|   stm32f401_d_e_wlcsp49 IBIS Model
[IBIS ver]   4.2
[File name]  stm32f401_d_e_wlcsp49.ibs
[File Rev]   1.0
[Date]   09-06-2015
[Source] Data Created at STMicroelectronics
[Notes]   File originated from ELDO simulations.
[Disclaimer]  This information is for modeling purpose only and is
   not guaranted. The information is subject to change without
   notice.
[Copyright] Copyright 2015 STMicroelectronics Inc.
[Component] stm32f401_d_e_wlcsp49
[Manufacturer] STMicroelectronics
[Package]
| variable   typ   min   max
R_pkg   0.0   NA   NA
L_pkg   0.0H   NA   NA
C_pkg   0.0F   NA   NA
[Pin]   signal_name   model_name   R_pin   L_pin   C_pin
A1 PA14 io8p_arsudq_ft
A2 PA15 io8p_arsudq_ft
A3 PB3 io8p_arsudq_i2cin_ft
A4 PB4 io8p_arsudq_i2cin_ft
A5 BOOT0 vpp_test_hv
A6 VSS gnd
A7 VDD power
B1 VSS gnd
B2 VDD power
B3 PA13 io8p_arsudq_ft
B4 PB5 io8p_ar3wsudq_ft
B5 PB8 io8p_arsudq_i2cin_ft
B6 PDR_ON io8p_arsudq_ft_v33
B7 VBAT power
C1 PA11 io8usb_lsfs_otg_ft
C2 PA10 io8usb_id_otg_ft
C3 PA12 io8usb_lsfs_otg_ft
C4 PB6 io8p_arsudq_i2cin_ft
C5 PB9 io8p_arsudq_i2cin_ft
C6 PC15-OSC32_OUT io8p_arsudq_ft
C7 PC14-OSC32_IN io8p_arwsudq_ft
D1 PA8 io8p_arsudq_i2cin_ft
D2 PA9 io8usb_vbus_otg_ft
D3 VSS gnd
D4 PB7 io8p_arsudq_i2cin_ft
D5 PC13-ANTI_TAMP io8p_arwsudq_ft_v33
D6 PH1-OSC_OUT io8p_arsudq_ft
D7 PH0-OSC_IN io8p_arsudq_ft
E1 PB15 io8p_arsudq_ft
E2 PB12 io8p_arsudq_ft
E3 PB10 io8p_arsudq_i2cin_ft
E4 PA3 io8p_arwsudq_ft
E5 PA2 io8p_arwsudq_ft
E6 VSS gnd
E7 NRST ioreset_ft_v33
F1 PB14 io8p_arsudq_ft
F2 VDD power
F3 PA7 io8p_arwsudq_ft
F4 PA6 io8p_ar3wsudq_ft
F5 PA5 io8p_ar3wsudq_ft
F6 PA0-WKUP io8p_arwsudq_ft_v33
F7 VDDA power
G1 PB13 io8p_arsudq_ft
G2 VCAP1 power
G3 PB2 io8p_arwsudq_ft
G4 PB1 io8p_ar3wsudq_ft
G5 PB0 io8p_ar3wsudq_ft
G6 PA4 io8p_ar3wsudq_ft
G7 PA1 io8p_arwsudq_ft
[Diff Pin]   inv_pin   vdiff   tdelay_typ  tdelay_min  tdelay_max
C1 C3 200mV   NA   NA   NA
[Model Selector] io8p_ar3wsudq_ft
io8p00_ar3wsudq_ft_pd_lv  "SPEED00 1P8V, PD=40kOhm"
io8p00_ar3wsudq_ft_pu_lv  "SPEED00 1P8V, PU=40kOhm"
io8p00_ar3wsudq_ft_lv  "SPEED00 1P8V"
io8p01_ar3wsudq_ft_pd_lv  "SPEED01 1P8V, PD=40kOhm"
io8p01_ar3wsudq_ft_pu_lv  "SPEED01 1P8V, PU=40kOhm"
io8p01_ar3wsudq_ft_lv  "SPEED01 1P8V"
io8p10_ar3wsudq_ft_pd_lv  "SPEED10 1P8V, PD=40kOhm"
io8p10_ar3wsudq_ft_pu_lv  "SPEED10 1P8V, PU=40kOhm"
io8p10_ar3wsudq_ft_lv  "SPEED10 1P8V"
io8p11_ar3wsudq_ft_pd_lv  "SPEED11 1P8V, PD=40kOhm"
io8p11_ar3wsudq_ft_pu_lv  "SPEED11 1P8V, PU=40kOhm"
io8p11_ar3wsudq_ft_lv  "SPEED11 1P8V"
io8p00_ar3wsudq_ft_pd  "SPEED00, PD=40kOhm"
io8p00_ar3wsudq_ft_pu  "SPEED00, PU=40kOhm"
io8p00_ar3wsudq_ft  "SPEED00"
io8p01_ar3wsudq_ft_pd  "SPEED01, PD=40kOhm"
io8p01_ar3wsudq_ft_pu  "SPEED01, PU=40kOhm"
io8p01_ar3wsudq_ft  "SPEED01"
io8p10_ar3wsudq_ft_pd  "SPEED10, PD=40kOhm"
io8p10_ar3wsudq_ft_pu  "SPEED10, PU=40kOhm"
io8p10_ar3wsudq_ft  "SPEED10"
io8p11_ar3wsudq_ft_pd  "SPEED11, PD=40kOhm"
io8p11_ar3wsudq_ft_pu  "SPEED11, PU=40kOhm"
io8p11_ar3wsudq_ft  "SPEED11"
[Model Selector] io8p_arsudq_ft
io8p00_arsudq_ft_pd_lv  "SPEED00 1P8V, PD=40kOhm"
io8p00_arsudq_ft_pu_lv  "SPEED00 1P8V, PU=40kOhm"
io8p00_arsudq_ft_lv  "SPEED00 1P8V"
io8p01_arsudq_ft_pd_lv  "SPEED01 1P8V, PD=40kOhm"
io8p01_arsudq_ft_pu_lv  "SPEED01 1P8V, PU=40kOhm"
io8p01_arsudq_ft_lv  "SPEED01 1P8V"
io8p10_arsudq_ft_pd_lv  "SPEED10 1P8V, PD=40kOhm"
io8p10_arsudq_ft_pu_lv  "SPEED10 1P8V, PU=40kOhm"
io8p10_arsudq_ft_lv  "SPEED10 1P8V"
io8p11_arsudq_ft_pd_lv  "SPEED11 1P8V, PD=40kOhm"
io8p11_arsudq_ft_pu_lv  "SPEED11 1P8V, PU=40kOhm"
io8p11_arsudq_ft_lv  "SPEED11 1P8V"
io8p00_arsudq_ft_pd  "SPEED00, PD=40kOhm"
io8p00_arsudq_ft_pu  "SPEED00, PU=40kOhm"
io8p00_arsudq_ft  "SPEED00"
io8p01_arsudq_ft_pd  "SPEED01, PD=40kOhm"
io8p01_arsudq_ft_pu  "SPEED01, PU=40kOhm"
io8p01_arsudq_ft  "SPEED01"
io8p10_arsudq_ft_pd  "SPEED10, PD=40kOhm"
io8p10_arsudq_ft_pu  "SPEED10, PU=40kOhm"
io8p10_arsudq_ft  "SPEED10"
io8p11_arsudq_ft_pd  "SPEED11, PD=40kOhm"
io8p11_arsudq_ft_pu  "SPEED11, PU=40kOhm"
io8p11_arsudq_ft  "SPEED11"
[Model Selector] io8p_arsudq_ft_v33
io8p00_arsudq_ft_v33_pd_lv  "SPEED00 1P8V, PD=40kOhm"
io8p00_arsudq_ft_v33_pu_lv  "SPEED00 1P8V, PU=40kOhm"
io8p00_arsudq_ft_v33_lv  "SPEED00 1P8V"
io8p01_arsudq_ft_v33_pd_lv  "SPEED01 1P8V, PD=40kOhm"
io8p01_arsudq_ft_v33_pu_lv  "SPEED01 1P8V, PU=40kOhm"
io8p01_arsudq_ft_v33_lv  "SPEED01 1P8V"
io8p10_arsudq_ft_v33_pd_lv  "SPEED10 1P8V, PD=40kOhm"
io8p10_arsudq_ft_v33_pu_lv  "SPEED10 1P8V, PU=40kOhm"
io8p10_arsudq_ft_v33_lv  "SPEED10 1P8V"
io8p11_arsudq_ft_v33_pd_lv  "SPEED11 1P8V, PD=40kOhm"
io8p11_arsudq_ft_v33_pu_lv  "SPEED11 1P8V, PU=40kOhm"
io8p11_arsudq_ft_v33_lv  "SPEED11 1P8V"
io8p00_arsudq_ft_v33_pd  "SPEED00, PD=40kOhm"
io8p00_arsudq_ft_v33_pu  "SPEED00, PU=40kOhm"
io8p00_arsudq_ft_v33  "SPEED00"
io8p01_arsudq_ft_v33_pd  "SPEED01, PD=40kOhm"
io8p01_arsudq_ft_v33_pu  "SPEED01, PU=40kOhm"
io8p01_arsudq_ft_v33  "SPEED01"
io8p10_arsudq_ft_v33_pd  "SPEED10, PD=40kOhm"
io8p10_arsudq_ft_v33_pu  "SPEED10, PU=40kOhm"
io8p10_arsudq_ft_v33  "SPEED10"
io8p11_arsudq_ft_v33_pd  "SPEED11, PD=40kOhm"
io8p11_arsudq_ft_v33_pu  "SPEED11, PU=40kOhm"
io8p11_arsudq_ft_v33  "SPEED11"
[Model Selector] io8p_arsudq_i2cin_ft
io8p00_arsudq_i2cin_ft_pd_lv  "SPEED00 1P8V, PD=40kOhm"
io8p00_arsudq_i2cin_ft_pu_lv  "SPEED00 1P8V, PU=40kOhm"
io8p00_arsudq_i2cin_ft_lv  "SPEED00 1P8V"
io8p01_arsudq_i2cin_ft_pd_lv  "SPEED01 1P8V, PD=40kOhm"
io8p01_arsudq_i2cin_ft_pu_lv  "SPEED01 1P8V, PU=40kOhm"
io8p01_arsudq_i2cin_ft_lv  "SPEED01 1P8V"
io8p10_arsudq_i2cin_ft_pd_lv  "SPEED10 1P8V, PD=40kOhm"
io8p10_arsudq_i2cin_ft_pu_lv  "SPEED10 1P8V, PU=40kOhm"
io8p10_arsudq_i2cin_ft_lv  "SPEED10 1P8V"
io8p11_arsudq_i2cin_ft_pd_lv  "SPEED11 1P8V, PD=40kOhm"
io8p11_arsudq_i2cin_ft_pu_lv  "SPEED11 1P8V, PU=40kOhm"
io8p11_arsudq_i2cin_ft_lv  "SPEED11 1P8V"
io8p00_arsudq_i2cin_ft_pd  "SPEED00, PD=40kOhm"
io8p00_arsudq_i2cin_ft_pu  "SPEED00, PU=40kOhm"
io8p00_arsudq_i2cin_ft  "SPEED00"
io8p01_arsudq_i2cin_ft_pd  "SPEED01, PD=40kOhm"
io8p01_arsudq_i2cin_ft_pu  "SPEED01, PU=40kOhm"
io8p01_arsudq_i2cin_ft  "SPEED01"
io8p10_arsudq_i2cin_ft_pd  "SPEED10, PD=40kOhm"
io8p10_arsudq_i2cin_ft_pu  "SPEED10, PU=40kOhm"
io8p10_arsudq_i2cin_ft  "SPEED10"
io8p11_arsudq_i2cin_ft_pd  "SPEED11, PD=40kOhm"
io8p11_arsudq_i2cin_ft_pu  "SPEED11, PU=40kOhm"
io8p11_arsudq_i2cin_ft  "SPEED11"
[Model Selector] io8p_arwsudq_ft
io8p00_arwsudq_ft_pd_lv  "SPEED00 1P8V, PD=40kOhm"
io8p00_arwsudq_ft_pu_lv  "SPEED00 1P8V, PU=40kOhm"
io8p00_arwsudq_ft_lv  "SPEED00 1P8V"
io8p01_arwsudq_ft_pd_lv  "SPEED01 1P8V, PD=40kOhm"
io8p01_arwsudq_ft_pu_lv  "SPEED01 1P8V, PU=40kOhm"
io8p01_arwsudq_ft_lv  "SPEED01 1P8V"
io8p10_arwsudq_ft_pd_lv  "SPEED10 1P8V, PD=40kOhm"
io8p10_arwsudq_ft_pu_lv  "SPEED10 1P8V, PU=40kOhm"
io8p10_arwsudq_ft_lv  "SPEED10 1P8V"
io8p11_arwsudq_ft_pd_lv  "SPEED11 1P8V, PD=40kOhm"
io8p11_arwsudq_ft_pu_lv  "SPEED11 1P8V, PU=40kOhm"
io8p11_arwsudq_ft_lv  "SPEED11 1P8V"
io8p00_arwsudq_ft_pd  "SPEED00, PD=40kOhm"
io8p00_arwsudq_ft_pu  "SPEED00, PU=40kOhm"
io8p00_arwsudq_ft  "SPEED00"
io8p01_arwsudq_ft_pd  "SPEED01, PD=40kOhm"
io8p01_arwsudq_ft_pu  "SPEED01, PU=40kOhm"
io8p01_arwsudq_ft  "SPEED01"
io8p10_arwsudq_ft_pd  "SPEED10, PD=40kOhm"
io8p10_arwsudq_ft_pu  "SPEED10, PU=40kOhm"
io8p10_arwsudq_ft  "SPEED10"
io8p11_arwsudq_ft_pd  "SPEED11, PD=40kOhm"
io8p11_arwsudq_ft_pu  "SPEED11, PU=40kOhm"
io8p11_arwsudq_ft  "SPEED11"
[Model Selector] io8p_arwsudq_ft_v33
io8p00_arwsudq_ft_v33_pd_lv  "SPEED00 1P8V, PD=40kOhm"
io8p00_arwsudq_ft_v33_pu_lv  "SPEED00 1P8V, PU=40kOhm"
io8p00_arwsudq_ft_v33_lv  "SPEED00 1P8V"
io8p01_arwsudq_ft_v33_pd_lv  "SPEED01 1P8V, PD=40kOhm"
io8p01_arwsudq_ft_v33_pu_lv  "SPEED01 1P8V, PU=40kOhm"
io8p01_arwsudq_ft_v33_lv  "SPEED01 1P8V"
io8p10_arwsudq_ft_v33_pd_lv  "SPEED10 1P8V, PD=40kOhm"
io8p10_arwsudq_ft_v33_pu_lv  "SPEED10 1P8V, PU=40kOhm"
io8p10_arwsudq_ft_v33_lv  "SPEED10 1P8V"
io8p11_arwsudq_ft_v33_pd_lv  "SPEED11 1P8V, PD=40kOhm"
io8p11_arwsudq_ft_v33_pu_lv  "SPEED11 1P8V, PU=40kOhm"
io8p11_arwsudq_ft_v33_lv  "SPEED11 1P8V"
io8p00_arwsudq_ft_v33_pd  "SPEED00, PD=40kOhm"
io8p00_arwsudq_ft_v33_pu  "SPEED00, PU=40kOhm"
io8p00_arwsudq_ft_v33  "SPEED00"
io8p01_arwsudq_ft_v33_pd  "SPEED01, PD=40kOhm"
io8p01_arwsudq_ft_v33_pu  "SPEED01, PU=40kOhm"
io8p01_arwsudq_ft_v33  "SPEED01"
io8p10_arwsudq_ft_v33_pd  "SPEED10, PD=40kOhm"
io8p10_arwsudq_ft_v33_pu  "SPEED10, PU=40kOhm"
io8p10_arwsudq_ft_v33  "SPEED10"
io8p11_arwsudq_ft_v33_pd  "SPEED11, PD=40kOhm"
io8p11_arwsudq_ft_v33_pu  "SPEED11, PU=40kOhm"
io8p11_arwsudq_ft_v33  "SPEED11"
[Model Selector] io8usb_id_otg_ft
io8p00_id_otg_ft_pd_lv  "SPEED00 1P8V, PD=14kOhm"
io8p00_id_otg_ft_pu_lv  "SPEED00 1P8V, PU=14kOhm"
io8p00_id_otg_ft_lv  "SPEED00 1P8V"
io8p01_id_otg_ft_pd_lv  "SPEED01 1P8V, PD=14kOhm"
io8p01_id_otg_ft_pu_lv  "SPEED01 1P8V, PU=14kOhm"
io8p01_id_otg_ft_lv  "SPEED01 1P8V"
io8p10_id_otg_ft_pd_lv  "SPEED10 1P8V, PD=14kOhm"
io8p10_id_otg_ft_pu_lv  "SPEED10 1P8V, PU=14kOhm"
io8p10_id_otg_ft_lv  "SPEED10 1P8V"
io8p11_id_otg_ft_pd_lv  "SPEED11 1P8V, PD=14kOhm"
io8p11_id_otg_ft_pu_lv  "SPEED11 1P8V, PU=14kOhm"
io8p11_id_otg_ft_lv  "SPEED11 1P8V"
io8p00_id_otg_ft_pd  "SPEED00, PD=14kOhm"
io8p00_id_otg_ft_pu  "SPEED00, PU=14kOhm"
io8p00_id_otg_ft  "SPEED00"
io8p01_id_otg_ft_pd  "SPEED01, PD=14kOhm"
io8p01_id_otg_ft_pu  "SPEED01, PU=14kOhm"
io8p01_id_otg_ft  "SPEED01"
io8p10_id_otg_ft_pd  "SPEED10, PD=14kOhm"
io8p10_id_otg_ft_pu  "SPEED10, PU=14kOhm"
io8p10_id_otg_ft  "SPEED10"
io8p11_id_otg_ft_pd  "SPEED11, PD=14kOhm"
io8p11_id_otg_ft_pu  "SPEED11, PU=14kOhm"
io8p11_id_otg_ft  "SPEED11"
[Model Selector] io8usb_lsfs_otg_ft
io8usb_ls_otg_ft_dpdn_pd  "LS USB DP/DN IO + PD=20kOhm"
io8usb_ls_otg_ft_dpdn_pupu2  "LS USB DP/DN IO + PU/PU2=2.2kOhm"
io8usb_ls_otg_ft_dpdn_pu2  "LS USB DP/DN IO + PU2=1.2kOhm"
io8usb_ls_otg_ft_dpdn_pu  "LS USB DP/DN IO + PU=1.2kOhm"
io8usb_ls_otg_ft_dpdn  "LS USB DP/DN IO"
io8usb_fs_otg_ft_dpdn_pd  "HS USB DP/DN IO + PD=20kOhm"
io8usb_fs_otg_ft_dpdn_pupu2  "HS USB DP/DN IO + PU/PU2=2.2kOhm"
io8usb_fs_otg_ft_dpdn_pu2  "HS USB DP/DN IO + PU2=1.2kOhm"
io8usb_fs_otg_ft_dpdn_pu  "HS USB DP/DN IO + PU=1.2kOhm"
io8usb_fs_otg_ft_dpdn  "HS USB DP/DN IO"
io8p00_lsfs_otg_ft_pd_lv  "SPEED00 1P8V, PD=40kOhm"
io8p00_lsfs_otg_ft_pu_lv  "SPEED00 1P8V, PU=40kOhm"
io8p00_lsfs_otg_ft_lv  "SPEED00 1P8V"
io8p01_lsfs_otg_ft_pd_lv  "SPEED01 1P8V, PD=40kOhm"
io8p01_lsfs_otg_ft_pu_lv  "SPEED01 1P8V, PU=40kOhm"
io8p01_lsfs_otg_ft_lv  "SPEED01 1P8V"
io8p10_lsfs_otg_ft_pd_lv  "SPEED10 1P8V, PD=40kOhm"
io8p10_lsfs_otg_ft_pu_lv  "SPEED10 1P8V, PU=40kOhm"
io8p10_lsfs_otg_ft_lv  "SPEED10 1P8V"
io8p11_lsfs_otg_ft_pd_lv  "SPEED11 1P8V, PD=40kOhm"
io8p11_lsfs_otg_ft_pu_lv  "SPEED11 1P8V, PU=40kOhm"
io8p11_lsfs_otg_ft_lv  "SPEED11 1P8V"
io8p00_lsfs_otg_ft_pd  "SPEED00, PD=40kOhm"
io8p00_lsfs_otg_ft_pu  "SPEED00, PU=40kOhm"
io8p00_lsfs_otg_ft  "SPEED00"
io8p01_lsfs_otg_ft_pd  "SPEED01, PD=40kOhm"
io8p01_lsfs_otg_ft_pu  "SPEED01, PU=40kOhm"
io8p01_lsfs_otg_ft  "SPEED01"
io8p10_lsfs_otg_ft_pd  "SPEED10, PD=40kOhm"
io8p10_lsfs_otg_ft_pu  "SPEED10, PU=40kOhm"
io8p10_lsfs_otg_ft  "SPEED10"
io8p11_lsfs_otg_ft_pd  "SPEED11, PD=40kOhm"
io8p11_lsfs_otg_ft_pu  "SPEED11, PU=40kOhm"
io8p11_lsfs_otg_ft  "SPEED11"
[Model Selector] io8usb_vbus_otg_ft
io8psenb_vbus_otg_ft  "VBUS PULSE, SENSE VB"
io8psenab_vbus_otg_ft  "VBUS PULSE, SENSE VA and VB"
io8psena_vbus_otg_ft  "VBUS PULSE, SENSE VA"
io8psen_vbus_otg_ft  "VBUS PULSE"
io8p00_vbus_otg_ft_pd_lv  "SPEED00 1P8V, PD=40kOhm"
io8p00_vbus_otg_ft_pu_lv  "SPEED00 1P8V, PU=40kOhm"
io8p00_vbus_otg_ft_lv  "SPEED00 1P8V"
io8p01_vbus_otg_ft_pd_lv  "SPEED01 1P8V, PD=40kOhm"
io8p01_vbus_otg_ft_pu_lv  "SPEED01 1P8V, PU=40kOhm"
io8p01_vbus_otg_ft_lv  "SPEED01 1P8V"
io8p10_vbus_otg_ft_pd_lv  "SPEED10 1P8V, PD=40kOhm"
io8p10_vbus_otg_ft_pu_lv  "SPEED10 1P8V, PU=40kOhm"
io8p10_vbus_otg_ft_lv  "SPEED10 1P8V"
io8p11_vbus_otg_ft_pd_lv  "SPEED11 1P8V, PD=40kOhm"
io8p11_vbus_otg_ft_pu_lv  "SPEED11 1P8V, PU=40kOhm"
io8p11_vbus_otg_ft_lv  "SPEED11 1P8V"
io8p00_vbus_otg_ft_pd  "SPEED00, PD=40kOhm"
io8p00_vbus_otg_ft_pu  "SPEED00, PU=40kOhm"
io8p00_vbus_otg_ft  "SPEED00"
io8p01_vbus_otg_ft_pd  "SPEED01, PD=40kOhm"
io8p01_vbus_otg_ft_pu  "SPEED01, PU=40kOhm"
io8p01_vbus_otg_ft  "SPEED01"
io8p10_vbus_otg_ft_pd  "SPEED10, PD=40kOhm"
io8p10_vbus_otg_ft_pu  "SPEED10, PU=40kOhm"
io8p10_vbus_otg_ft  "SPEED10"
io8p11_vbus_otg_ft_pd  "SPEED11, PD=40kOhm"
io8p11_vbus_otg_ft_pu  "SPEED11, PU=40kOhm"
io8p11_vbus_otg_ft  "SPEED11"
[Model Selector] ioreset_ft_v33
ioreset_ft_v33_pu_lv  "ioreset 1P8V + PU=40kOhm"
ioreset_ft_v33_nopu_lv  "ioreset 1P8V"
ioreset_ft_v33_pu  "ioreset + PU=40kOhm"
ioreset_ft_v33_nopu  "ioreset"
[Model Selector] vpp_test_hv
vpp_test_hv_2p4  "Input Buffer 1P8V"
vpp_test_hv_3p3  "Input Buffer"
| Models and submodels in the file (236): io8p00_ar3wsudq_ft_pd_lv (I/O), io8p00_ar3wsudq_ft_pu_lv (I/O), io8p00_ar3wsudq_ft_lv (I/O), io8p01_ar3wsudq_ft_pd_lv (I/O), io8p01_ar3wsudq_ft_pu_lv (I/O), io8p01_ar3wsudq_ft_lv (I/O), io8p10_ar3wsudq_ft_pd_lv (I/O), io8p10_ar3wsudq_ft_pu_lv (I/O), io8p10_ar3wsudq_ft_lv (I/O), io8p11_ar3wsudq_ft_pd_lv (I/O), io8p11_ar3wsudq_ft_pu_lv (I/O), io8p11_ar3wsudq_ft_lv (I/O), io8p00_ar3wsudq_ft_pd (I/O), io8p00_ar3wsudq_ft_pu (I/O), io8p00_ar3wsudq_ft (I/O), io8p01_ar3wsudq_ft_pd (I/O), io8p01_ar3wsudq_ft_pu (I/O), io8p01_ar3wsudq_ft (I/O), io8p10_ar3wsudq_ft_pd (I/O), io8p10_ar3wsudq_ft_pu (I/O), io8p10_ar3wsudq_ft (I/O), io8p11_ar3wsudq_ft_pd (I/O), io8p11_ar3wsudq_ft_pu (I/O), io8p11_ar3wsudq_ft (I/O), io8p00_arsudq_ft_pd_lv (I/O), io8p00_arsudq_ft_pu_lv (I/O), io8p00_arsudq_ft_lv (I/O), io8p01_arsudq_ft_pd_lv (I/O), io8p01_arsudq_ft_pu_lv (I/O), io8p01_arsudq_ft_lv (I/O), io8p10_arsudq_ft_pd_lv (I/O), io8p10_arsudq_ft_pu_lv (I/O), io8p10_arsudq_ft_lv (I/O), io8p11_arsudq_ft_pd_lv (I/O), io8p11_arsudq_ft_pu_lv (I/O), io8p11_arsudq_ft_lv (I/O), io8p00_arsudq_ft_pd (I/O), io8p00_arsudq_ft_pu (I/O), io8p00_arsudq_ft (I/O), io8p01_arsudq_ft_pd (I/O), io8p01_arsudq_ft_pu (I/O), io8p01_arsudq_ft (I/O), io8p10_arsudq_ft_pd (I/O), io8p10_arsudq_ft_pu (I/O), io8p10_arsudq_ft (I/O), io8p11_arsudq_ft_pd (I/O), io8p11_arsudq_ft_pu (I/O), io8p11_arsudq_ft (I/O), io8p00_arsudq_ft_v33_pd_lv (I/O), io8p00_arsudq_ft_v33_pu_lv (I/O), io8p00_arsudq_ft_v33_lv (I/O), io8p01_arsudq_ft_v33_pd_lv (I/O), io8p01_arsudq_ft_v33_pu_lv (I/O), io8p01_arsudq_ft_v33_lv (I/O), io8p10_arsudq_ft_v33_pd_lv (I/O), io8p10_arsudq_ft_v33_pu_lv (I/O), io8p10_arsudq_ft_v33_lv (I/O), io8p11_arsudq_ft_v33_pd_lv (I/O), io8p11_arsudq_ft_v33_pu_lv (I/O), io8p11_arsudq_ft_v33_lv (I/O), io8p00_arsudq_ft_v33_pd (I/O), io8p00_arsudq_ft_v33_pu (I/O), io8p00_arsudq_ft_v33 (I/O), io8p01_arsudq_ft_v33_pd (I/O), io8p01_arsudq_ft_v33_pu (I/O), io8p01_arsudq_ft_v33 (I/O), io8p10_arsudq_ft_v33_pd (I/O), io8p10_arsudq_ft_v33_pu (I/O), io8p10_arsudq_ft_v33 (I/O), io8p11_arsudq_ft_v33_pd (I/O), io8p11_arsudq_ft_v33_pu (I/O), io8p11_arsudq_ft_v33 (I/O), io8p00_arsudq_i2cin_ft_pd_lv (I/O), io8p00_arsudq_i2cin_ft_pu_lv (I/O), io8p00_arsudq_i2cin_ft_lv (I/O), io8p01_arsudq_i2cin_ft_pd_lv (I/O), io8p01_arsudq_i2cin_ft_pu_lv (I/O), io8p01_arsudq_i2cin_ft_lv (I/O), io8p10_arsudq_i2cin_ft_pd_lv (I/O), io8p10_arsudq_i2cin_ft_pu_lv (I/O)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
